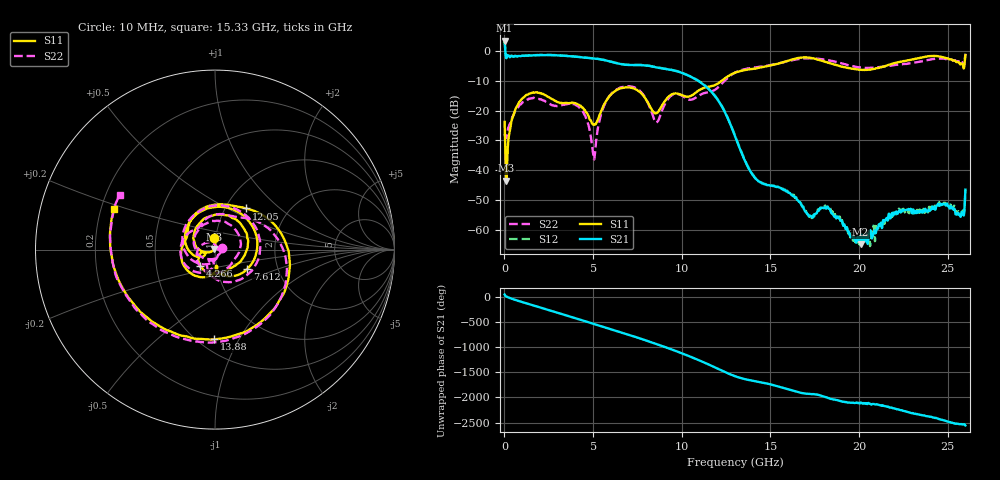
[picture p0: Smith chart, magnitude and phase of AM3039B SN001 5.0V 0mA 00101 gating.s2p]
!Agilent Technologies,E8364B,MY43040894,A.07.50.67
!Agilent E8364B: A.07.50.67
!Date: Tuesday, June 28, 2016 08:04:24
!Correction: S11(Full 2 Port(1,2))
!S21(Full 2 Port(1,2))
!S12(Full 2 Port(1,2))
!S22(Full 2 Port(1,2))
!S2P File: Measurements: S11, S21, S12, S22:
# Hz S  dB  R 50
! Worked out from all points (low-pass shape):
!   1601 points, 10 MHz to 26 GHz, reference 50 ohm
!   highest |S21| = 3.59 dB at 10 MHz (marker M1); lowest = -65.0 dB at 20.09 GHz (marker M2)
!   |S21| within 3 dB of the highest: start of sweep to 44.49 MHz
!   lowest |S11| = -43.6 dB at 107.5 MHz (marker M3), VSWR 1.01, Z = 49.5 + j0.406 ohm
!   |S11| at or under -10 dB: start of sweep to 12.24 GHz
!   |S22| runs from -36.4 to -0.8 dB; largest |S21 - S12| = 0.025
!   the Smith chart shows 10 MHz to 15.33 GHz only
!   S11 on the Smith chart (normalised r, x): 10 MHz: 0.98, +0.13; 4.266 GHz: 0.83, -0.15; 7.612 GHz: 1.39, -0.32; 12.05 GHz: 1.25, +0.62; 13.88 GHz: 0.60, -0.79; 15.33 GHz: 0.25, +0.18
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1e7  -23.78 95.3  3.59 40.5  3.65 41.4  -27.75 15.2
1.074625e8  -43.55 141.8  -2.32 3.5  -2.25 3.5  -29.14 -59.1
7.572125e8  -18.02 157.4  -1.63 -82.0  -1.58 -81.8  -18.95 174.2
1.601888e9  -13.90 71.0  -1.34 -172.6  -1.29 -172.4  -15.75 75.9
2.609e9  -15.85 -18.5  -1.28 80.6  -1.22 80.9  -17.93 -16.3
3.404944e9  -17.44 -65.7  -1.53 -4.8  -1.47 -4.6  -17.94 -69.4
4.265862e9  -18.22 -132.1  -1.97 -98.0  -1.91 -97.8  -19.27 -159.5
4.347081e9  -18.74 -140.0  -2.03 -106.9  -1.99 -106.7  -19.75 -168.8
5.744044e9  -16.62 -178.7  -3.12 97.7  -3.06 98.0  -16.75 -158.9
7.612075e9  -13.58 -31.2  -4.62 -106.5  -4.57 -106.2  -13.16 -48.6
8.684162e9  -20.25 -82.4  -5.54 124.4  -5.46 124.8  -23.27 -98.1
1.204662e10  -10.83 52.8  -16.46 7.1  -16.31 7.6  -12.15 45.2
1.3005e10  -7.21 -19.2  -28.58 -140.1  -28.39 -140.0  -7.19 -25.9
1.388216e10  -6.02 -90.5  -40.54 138.1  -40.47 137.1  -5.66 -100.1
1.532786e10  -4.35 158.3  -45.65 26.8  -45.57 26.5  -4.25 150.2
1.734208e10  -2.30 -23.2  -55.73 -136.1  -56.13 -134.5  -2.38 -15.6
2.008728e10  -6.20 118.7  -65.01 51.7  -62.38 51.9  -5.45 128.1
2.167916e10  -4.52 12.8  -54.71 -31.1  -55.32 -27.6  -4.92 18.2
2.309237e10  -2.64 -93.2  -53.73 -164.7  -53.76 -154.6  -3.85 -83.8
2.41807e10  -1.56 178.6  -52.93 117.7  -52.36 121.9  -2.60 -166.9
2.513908e10  -2.69 96.5  -52.62 30.5  -51.56 29.4  -2.76 112.7
2.6e10  -1.27 -25.0  -46.59 -37.8  -46.60 -35.4  -0.83 2.8
